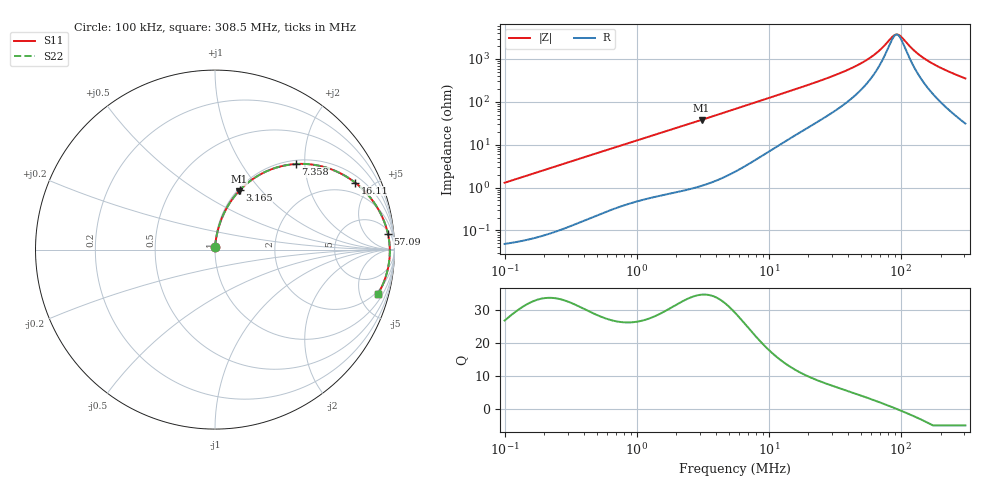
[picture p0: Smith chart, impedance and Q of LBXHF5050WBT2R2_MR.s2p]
! LBXHF5050WBT2R2_MR  S-PARAMETER MODEL  ( General Type )
! Model Generated by TAIYO YUDEN Corporation (http://www.ty-top.com)
! Version 1.0
! TAIYO YUDEN Control No. 210719NI43SB-FBB
! Copyright(c) 2021 TAIYO YUDEN CO.,LTD. All Rights Reserved.
! Product Description (link to TY-COMPAS)
! https://ds.yuden.co.jp/TYCOMPAS/or/detail?pn=LBXHF5050WBT2R2NMR&u=M
! Products Name : Inductors
! Characteristics :
!  Inductance : 2.2 uH , SRF(min) : 65 MHz , DC Resistance(max) : 0.036 Ohm
!  Rated Current : Saturation :3200 mA , Temp Rise : 2100 mA
!  Case Size : 5.0 x 5.0 / 0.197 x 0.197 [mm/inch] , Thickness : 2.2 / 0.087 [mm/inch]
!  (Conditions: Temperature = 25 degC , DC Bias Current/Voltage = 0A / 0V)
! External Node Assignments :
!  1  o---GGG---o  2
! GND o---------o GND
! Frequency Range : 0.1MHz  -  308.54851MHz  [ 402 STEP ]
# MHz S RI R 50
! Freq[MHz].  S11 Real  S11 Imag  S21 Real  S21 Imag  S12 Real  S12 Imag  S22 Real  S22 Imag
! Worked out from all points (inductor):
!   401 points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, 100 kHz to 308.5 MHz, reference 50 ohm
!   read as one part in series: L = 2.06 uH near 104.1 kHz
!   highest Q = 34.5 at 3.102 MHz (marker M1), where L = 1.94 uH
!   self-resonance near 93.03 MHz
!   S11 on the Smith chart (normalised r, x): 100 kHz: 1.00, +0.03; 3.165 MHz: 1.02, +0.77; 7.358 MHz: 1.08, +1.80; 16.11 MHz: 1.34, +3.98; 57.09 MHz: 7, +19; 308.5 MHz: 1.62, -7.02
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0.1  0.000651 0.0129  0.9993 -0.0129  0.9993 -0.0129  0.000651 0.0129
0.384115  0.004 0.0488  0.996 -0.0488  0.996 -0.0488  0.004 0.0488
0.807652  0.0139 0.0995  0.9861 -0.0995  0.9861 -0.0995  0.0139 0.0995
1.475446  0.0377 0.1739  0.9623 -0.1739  0.9623 -0.1739  0.0377 0.1739
3.102314  0.1327 0.3251  0.8673 -0.3251  0.8673 -0.3251  0.1327 0.3251
3.165258  0.1372 0.3299  0.8628 -0.3299  0.8628 -0.3299  0.1372 0.3299
5.667415  0.3306 0.4533  0.6694 -0.4533  0.6694 -0.4533  0.3306 0.4533
7.358479  0.4512 0.4768  0.5488 -0.4768  0.5488 -0.4768  0.4512 0.4768
10.35343  0.6127 0.4591  0.3873 -0.4591  0.3873 -0.4591  0.6127 0.4591
16.10635  0.7804 0.3733  0.2196 -0.3733  0.2196 -0.3733  0.7804 0.3733
21.33651  0.853 0.3044  0.147 -0.3044  0.147 -0.3044  0.853 0.3044
38.20317  0.9378 0.1686  0.0622 -0.1686  0.0622 -0.1686  0.9378 0.1686
57.09072  0.9635 0.0881  0.0365 -0.0881  0.0365 -0.0881  0.9635 0.0881
68.40302  0.9696 0.0548  0.0304 -0.0548  0.0304 -0.0548  0.9696 0.0548
81.95682  0.973 0.0224  0.027 -0.0224  0.027 -0.0224  0.973 0.0224
88.81336  0.9738 0.00821  0.0262 -0.00821  0.0262 -0.00821  0.9738 0.00821
96.24353  0.9741 -0.00603  0.0259 0.00603  0.0259 0.00603  0.9741 -0.00603
102.2213  0.974 -0.0167  0.026 0.0167  0.026 0.0167  0.974 -0.0167
127.4964  0.9715 -0.0568  0.0285 0.0568  0.0285 0.0568  0.9715 -0.0568
155.8587  0.9657 -0.0951  0.0343 0.0951  0.0343 0.0951  0.9657 -0.0951
214.9334  0.9475 -0.1627  0.0525 0.1627  0.0525 0.1627  0.9475 -0.1627
308.5485  0.9065 -0.2501  0.0935 0.2501  0.0935 0.2501  0.9065 -0.2501
